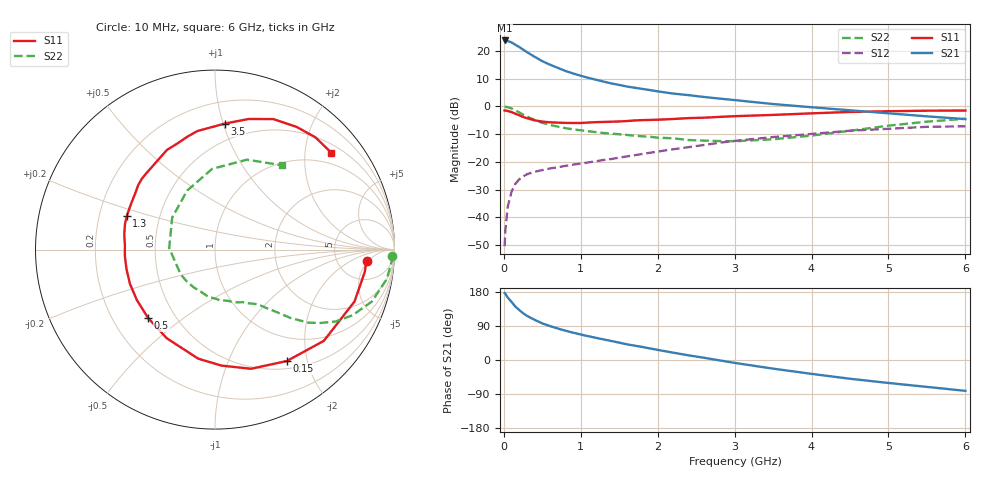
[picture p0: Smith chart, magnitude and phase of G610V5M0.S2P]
! SIEMENS Small Signal Semiconductors
! BFG193
! Si NPN RF Bipolar Junction Transistor in SOT223
! VCE = 10 V  IC = 5 mA
! Common Emitter S-Parameters:  August  1996
# GHz  S  MA  R  50
!  f  S11  S21  S12  S22
! GHz  MAG  ANG  MAG  ANG  MAG  ANG  MAG  ANG
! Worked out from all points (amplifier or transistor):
!   36 points, 10 MHz to 6 GHz, reference 50 ohm
!   highest |S21| = 23.8 dB at 10 MHz (marker M1)
!   |S21| within 3 dB of that: start of sweep to 235 MHz
!   unconditionally stable (mu >= 1): 1.176 GHz to 2.598 GHz
!   at 250 MHz: K = 0.33, MSG = 22.9 dB, |S12| = -25.3 dB
!   at 1.4 GHz: K = 1.07, MAG = 12.0 dB, |S12| = -19.0 dB
!   at 6 GHz: K = 0.86, MSG = 1.3 dB, |S12| = -7.2 dB
!   S11 on the Smith chart (normalised r, x): 10 MHz: 10, -5; 150 MHz: 0.61, -1.67; 500 MHz: 0.35, -0.38; 1.3 GHz: 0.32, +0.17; 3.5 GHz: 0.36, +1.01; 6 GHz: 0.70, +2.61
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0.01  0.8469 -4.3  15.57 176.7  0.003 89.5  0.9887 -2.0
0.02  0.8434 -8.6  15.52 174.7  0.0058 82.2  0.9866 -3.9
0.05  0.8295 -20.4  15.2 165.0  0.0154 78.8  0.9713 -9.7
0.1  0.7913 -40.0  14.35 153.4  0.0289 70.4  0.921 -18.3
0.15  0.7386 -57.2  12.99 140.9  0.0401 62.0  0.8492 -25.5
0.2  0.6936 -73.2  11.87 131.9  0.0484 55.9  0.7824 -30.8
0.25  0.6473 -86.8  10.68 123.4  0.0544 50.8  0.7118 -35.1
0.3  0.6149 -98.7  9.586 116.6  0.0596 47.7  0.6594 -38.1
0.4  0.5625 -118.5  7.891 106.1  0.0662 43.0  0.5689 -42.1
0.5  0.5332 -134.3  6.584 96.6  0.071 40.4  0.5059 -44.6
0.6  0.5181 -147.3  5.686 89.5  0.0761 39.4  0.4645 -46.7
0.7  0.5108 -158.1  4.98 83.1  0.0798 38.8  0.4328 -48.7
0.9  0.5035 -175.8  3.95 72.1  0.0891 38.8  0.3864 -52.1
1.1  0.5126 170.5  3.285 62.7  0.0977 39.6  0.3566 -57.2
1.3  0.5258 159.0  2.809 54.2  0.1081 39.9  0.3312 -62.1
1.6  0.5457 144.0  2.292 41.4  0.1254 39.3  0.3059 -72.2
2.2  0.5935 121.8  1.711 19.4  0.1685 34.7  0.2664 -97.6
2.8  0.6478 103.7  1.389 -0.9  0.221 26.1  0.2372 -132.0
3.5  0.704 85.6  1.107 -22.8  0.2802 11.7  0.2554 178.1
4.5  0.7965 65.9  0.853 -49.5  0.3648 -8.8  0.3638 115.2
5.5  0.8392 48.2  0.663 -71.0  0.4295 -34.9  0.5318 70.4
6  0.8436 39.7  0.592 -81.4  0.4383 -49.9  0.6004 51.5
